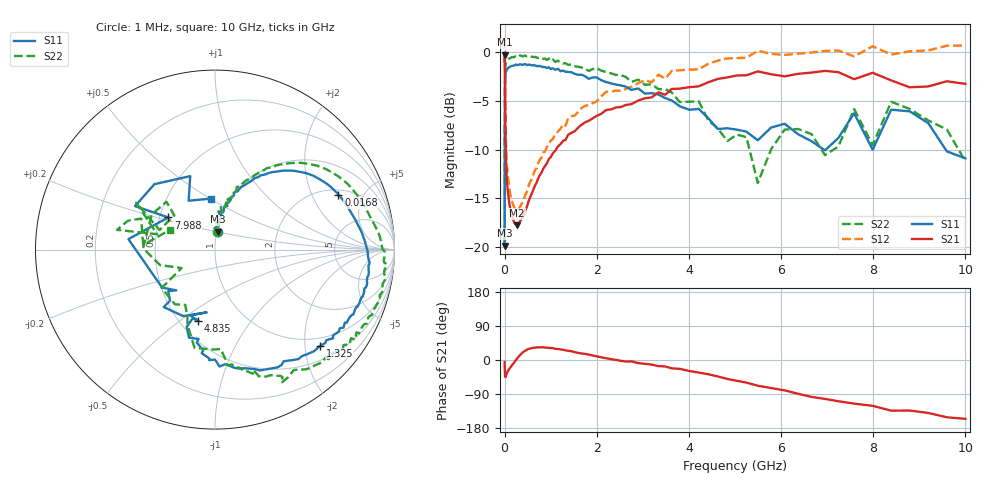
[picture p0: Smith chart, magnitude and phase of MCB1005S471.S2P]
!Agilent Technologies,E5071C,MY46111244,A.11.31
!Date: Tue May 07 14:52:30 2019
!Data & Calibration Information:
!Freq	S11:SOLT2(ON)	S21:SOLT2(ON)	S12:SOLT2(ON)	S22:SOLT2(ON)
# Hz S dB R 50
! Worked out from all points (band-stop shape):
!   201 points, 1 MHz to 10 GHz, reference 50 ohm
!   highest |S21| = -0.25 dB at 1.212 MHz (marker M1); lowest = -17.8 dB at 275.4 MHz (marker M2)
!   |S21| within 3 dB of the highest: 4.338 GHz to 8.593 GHz (4.255 GHz wide, 65.8 % of centre); 9.393 GHz to end of sweep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
!   lowest |S11| = -19.9 dB at 1 MHz (marker M3), VSWR 1.23, Z = 50.6 + j10.2 ohm
!   |S11| at or under -10 dB: start of sweep to 3.278 MHz; 6.926 GHz to 6.973 GHz (46.69 MHz wide, 0.672 % of centre); 9.571 GHz to end of sweep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
!   |S22| runs from -19.9 to -0.3 dB; largest |S21 - S12| = 0.49
!   S11 on the Smith chart (normalised r, x): 1 MHz: 1.01, +0.20; 16.8 MHz: 2.27, +3.20; 1.325 GHz: 0.81, -2.34; 4.835 GHz: 0.62, -0.59; 7.988 GHz: 0.56, +0.22; 10 GHz: 0.81, +0.50
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1000000  -19.87 81.0  -0.35 -5.3  1.09 -6.2  -19.94 82.7
1212171  -18.46 91.2  -0.25 -6.8  1.22 -7.8  -17.96 85.9
4810209  -7.11 61.6  -1.43 -26.0  0.08 -26.8  -6.23 60.6
1.680428e7  -2.47 24.0  -7.48 -45.2  -5.94 -45.7  -1.53 23.1
2.206931e7  -2.21 18.3  -9.13 -43.9  -7.60 -44.4  -1.29 17.5
1.047129e8  -1.52 2.4  -15.56 -23.4  -14.05 -23.3  -0.64 1.6
2.754229e8  -1.32 -6.1  -17.80 4.2  -16.27 4.8  -0.43 -6.6
4.810209e8  -1.31 -14.6  -15.94 26.8  -14.38 27.8  -0.43 -15.3
1.324842e9  -2.00 -42.4  -9.01 25.4  -7.54 29.1  -1.12 -44.0
2.206931e9  -3.07 -71.5  -5.93 4.5  -4.06 10.3  -2.03 -62.6
3.484689e9  -4.70 -97.3  -4.36 -17.0  -2.71 -8.2  -3.78 -84.1
4.83488e9  -7.81 -103.1  -2.58 -50.0  -0.63 -37.7  -9.13 -118.2
5.248075e9  -8.16 -110.4  -2.36 -59.7  -0.56 -46.8  -8.72 -144.3
5.495409e9  -9.05 -97.6  -1.97 -67.9  0.16 -55.1  -13.44 -151.0
6.078392e9  -7.35 -131.7  -2.47 -80.1  -0.27 -66.1  -7.95 178.9
6.661376e9  -9.15 -138.4  -2.09 -97.3  -0.02 -81.1  -8.42 135.4
7.24436e9  -8.81 -144.4  -2.04 -108.9  0.18 -89.6  -9.70 160.5
7.585776e9  -6.27 173.1  -2.77 -115.1  -0.42 -99.6  -5.85 149.3
7.988146e9  -10.01 145.4  -2.11 -121.0  0.62 -103.9  -9.54 165.1
8.390517e9  -5.90 151.4  -2.89 -133.7  -0.23 -114.5  -5.09 168.6
9.195259e9  -7.29 108.6  -3.51 -139.8  0.19 -122.9  -7.01 157.2
1e10  -10.91 94.8  -3.25 -155.3  0.68 -135.6  -11.21 156.5
